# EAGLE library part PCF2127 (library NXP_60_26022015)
Integrated RTC, TCXO and quartz crystal The PCF2127AT is a CMOS2 Real Time Clock (RTC) and calendar with an integrated Temperature Compensated Crystal (Xtal) Oscillator (TCXO) and a 32.768 kHz quartz crystal optimized for very high accuracy and very low power consumption. The PCF2127AT has 512 bytes of general purpose static RAM, a selectable I2C-bus or SPI-bus, a backup battery switch-over circuit, a programmable watchdog function, a timestamp function, and many other features. AAL Eindhoven MK
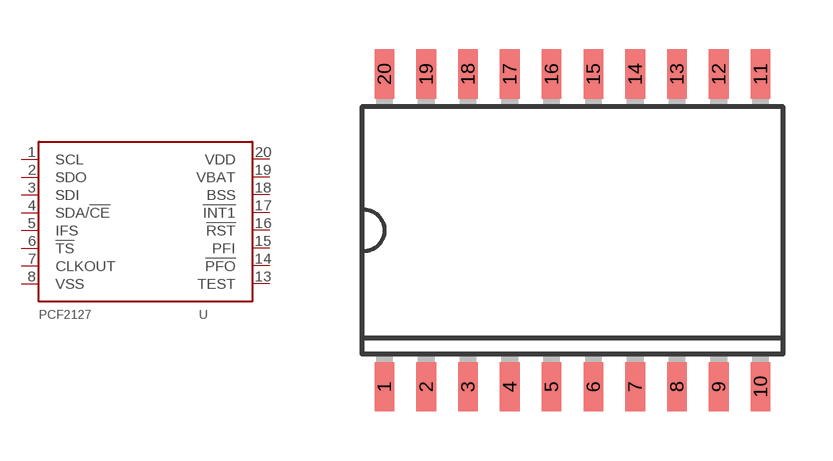
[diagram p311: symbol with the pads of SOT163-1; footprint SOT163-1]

Designator prefix U

## PCF2127AT  [SOT163-1]
1  SCL
2  SDO  out
3  SDI  in
4  SDA/!CE  in
5  IFS  in
6  !TS!  in
7  CLKOUT  out
8  VSS  pwr
13  TEST  nc
14  !PFO  out
15  PFI  in
16  !RST  in
17  !INT1!  out
18  BSS  out
19  VBAT  pwr
20  VDD  pwr

## Footprint SOT163-1 (pad centres in mm)
SOT163-1 SO20: plastic small outline package; 20 leads; body width 7.5 mm JEDEC: MS-013 IEC: 075E04
smd 0.6 x 1.5: 1 -5.715,-4.75; 2 -4.445,-4.75; 3 -3.175,-4.75; 4 -1.905,-4.75; 5 -0.635,-4.75; 6 0.635,-4.75; 7 1.905,-4.75; 8 3.175,-4.75; 9 4.445,-4.75; 10 5.715,-4.75; 11 5.715,4.75; 12 4.445,4.75; 13 3.175,4.75; 14 1.905,4.75; 15 0.635,4.75; 16 -0.635,4.75; 17 -1.905,4.75; 18 -3.175,4.75; 19 -4.445,4.75; 20 -5.715,4.75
